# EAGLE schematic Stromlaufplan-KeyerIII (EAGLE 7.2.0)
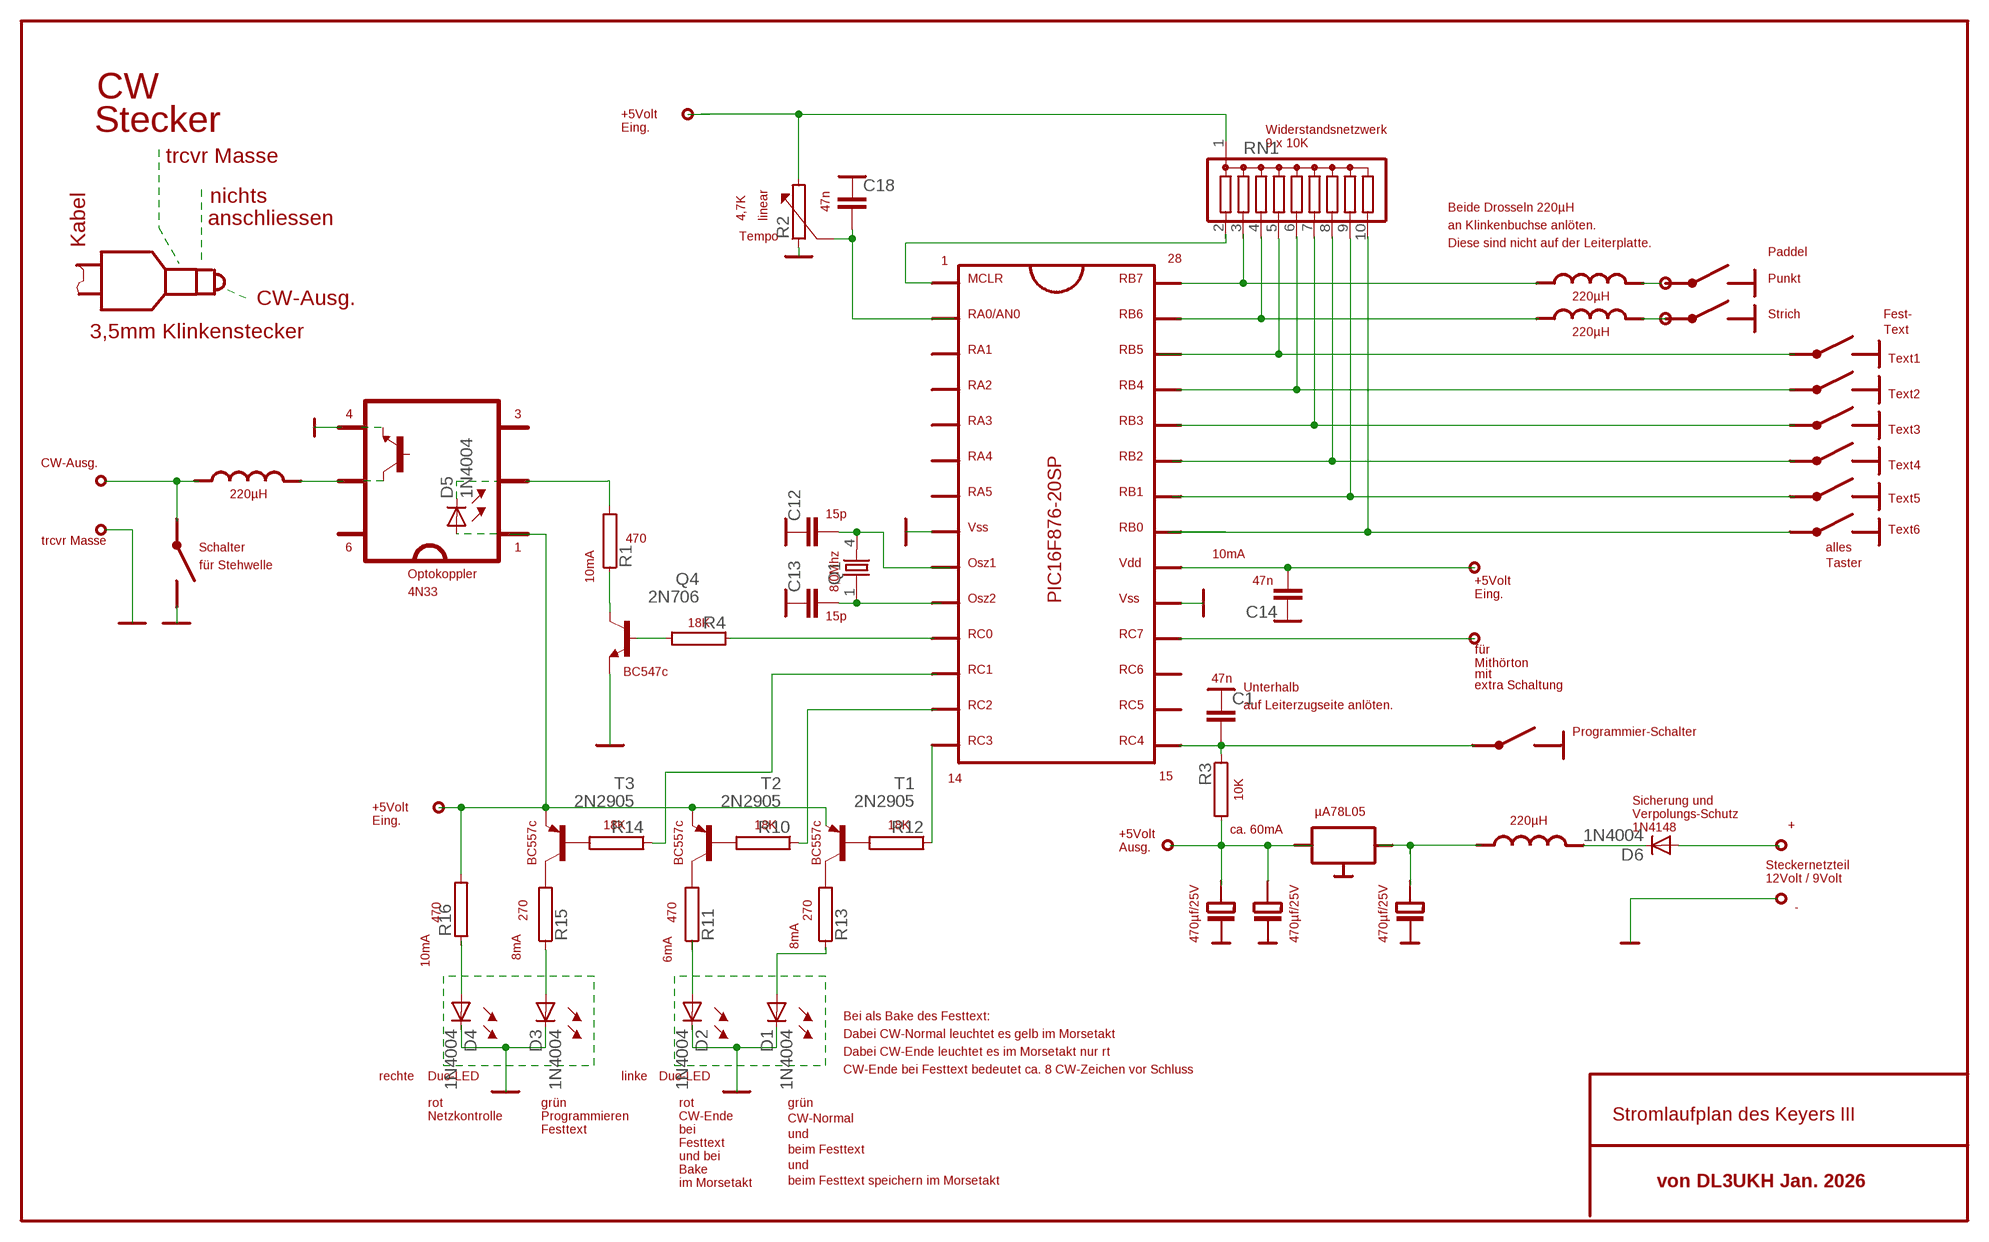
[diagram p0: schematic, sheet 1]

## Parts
C1  C2,5-3  [C2.5-3]
C12  C2,5-3  [C2.5-3]
C13  C2,5-3  [C2.5-3]
C14  C2,5-3  [C2.5-3]
C18  C2,5-3  [C2.5-3]
D1  1N4004  [DO41-10]
D2  1N4004  [DO41-10]
D3  1N4004  [DO41-10]
D4  1N4004  [DO41-10]
D5  1N4004  [DO41-10]
D6  1N4004  [DO41-10]
Q1  86SMX  [86SMX]
Q4  2N706  [TO18]
R1  RHS10  [HS10]
R2  RHS10  [HS10]
R3  RHS10  [HS10]
R4  RHS10  [HS10]
R10  RHS10  [HS10]
R11  RHS10  [HS10]
R12  RHS10  [HS10]
R13  RHS10  [HS10]
R14  RHS10  [HS10]
R15  RHS10  [HS10]
R16  RHS10  [HS10]
RN1  G09R  [SIL10]
T1  2N2905  [TO5]
T2  2N2905  [TO5]
T3  2N2905  [TO5]

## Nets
N$4: RN1.5
N$8: RN1.9
N$13: C14.2
N$17: C12.2 Q1.4
N$18: C13.2 Q1.1
N$22: C18.2
N$25: D6.A
N$28: D1.A
N$29: D2.A
N$30: D2.C
N$33: Q4.2(B)
N$34: R1.2
N$36: Q4.1(E)
N$37: R3.1
N$38: R4.1
N$40: Q4.3(C) R1.1
N$41: R10.2 T2.2(B)
N$43: R12.2 T1.2(B)
N$44: R13.2 T1.3(C)
N$45: R11.2 T2.3(C)
N$47: R14.2 T3.2(B)
N$48: D5.A
N$50: R15.2 T3.3(C)
N$51: D3.A R15.1
N$52: R12.1
N$53: R10.1
N$55: R14.1
N$57: D4.A
N$58: D4.C
N$60: D5.C
N$64: R16.2 T1.1(E) T2.1(E) T3.1(E)
N$83: R2.1
Unconnected: C1.1 C1.2 C12.1 C13.1 C14.1 C18.1 D1.C D3.C D6.C R2.2 R3.2 R4.2 R11.1 R13.1 R16.1 RN1.1 RN1.2 RN1.3 RN1.4 RN1.6 RN1.7 RN1.8 RN1.10

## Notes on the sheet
- CW
- +5Volt
- Stecker | Eing. | Widerstandsnetzwerk
- 9 x 10K
- trcvr Masse
- nichts
- 47n | Beide Drosseln 220µH
- 4,7K | linear
- anschliessen
- an Klinkenbuchse anlöten.
- Tempo
- Kabel | Diese sind nicht auf der Leiterplatte.
- Paddel
- 1 | 28
- MCLR | RB7 | Punkt
- 220µH
- CW-Ausg.
- RA0/AN0 | RB6 | Strich | Fest-
- 220µH | Text
- 3,5mm Klinkenstecker
- RA1 | RB5
- Text1
- RA2 | RB4
- Text2
- 4 | 3
- RA3 | RB3
- Text3
- RA4 | RB2
- CW-Ausg. | Text4
- 220µH | RA5 | RB1
- Text5
- 15p
- Vss | RB0 | Text6
- trcvr Masse | 470
- Schalter | 6 | 1 | alles
- 10mA
- für Stehwelle | Osz1 | Vdd | Taster
- Optokoppler
- 10mA | 47n | +5Volt
- 8,0Mhz
- 4N33 | Eing.
- Osz2 | PIC16F876-20SP | Vss
- 15p
- 18K
- RC0 | RC7
- für
- BC547c | Mithörton
- RC1 | RC6 | 47n
- mit
- Unterhalb | extra Schaltung
- RC2 | RC5 | auf Leiterzugseite anlöten.
- Programmier-Schalter
- RC3 | RC4
- 14 | 15
- 10K
- Sicherung und
- +5Volt
- µA78L05 | Verpolungs-Schutz
- Eing. | 220µH
- 18K | 18K | 18K | 1N4148 | +
- ca. 60mA
- +5Volt
- Ausg.
- BC557c | BC557c | BC557c
- Steckernetzteil
- 12Volt / 9Volt
- -
- 470 | 270 | 470 | 8mA | 270
- 10mA | 8mA | 6mA
- 470µf/25V | 470µf/25V | 470µf/25V
- Bei als Bake des Festtext:
- Dabei CW-Normal leuchtet es gelb im Morsetakt
- Dabei CW-Ende leuchtet es im Morsetakt nur rt
- CW-Ende bei Festtext bedeutet ca. 8 CW-Zeichen vor Schluss
- rechte | Duo-LED | linke | Duo-LED
- rot | grün | rot | grün
- Netzkontrolle | Programmieren | CW-Ende | CW-Normal | Stromlaufplan des Keyers III
- Festtext | bei
- und
- Festtext
- beim Festtext
- und bei
- und
- Bake
- im Morsetakt | beim Festtext speichern im Morsetakt | von DL3UKH Jan. 2026

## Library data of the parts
C1 C12-C14 C18 = capacitor-wima:C: CAPACITOR
D1-D6 = diode:1N4004: DIODE
Q1 = crystal:86SMX: CRYSTAL
Q4 = transistor-npn:2N706: NPN Transistor
R1-R4 R10-R16 = resistor-power:R: Power Resitor
RN1 = resistor-sil:G09R: SIL RESISTOR; OC_FARNELL: unknown; OC_NEWARK: unknown
T1-T3 = transistor-pnp:2N2905: PNP Transistor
